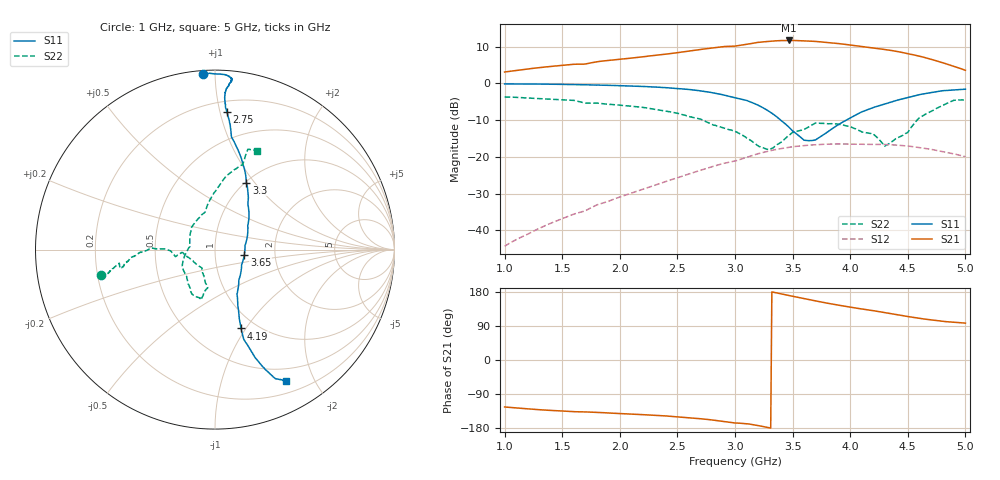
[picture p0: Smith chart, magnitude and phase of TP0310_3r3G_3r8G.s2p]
! Created Fri Jul 02 06:30:30 2021
# hz S ri R 50
! 2 Port Network Data from SP1.SP block
! freq  reS11  imS11  reS21  imS21  reS12  imS12  reS22  imS22
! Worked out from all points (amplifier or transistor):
!   401 points, 1 GHz to 5 GHz, reference 50 ohm
!   highest |S21| = 11.7 dB at 3.47 GHz (marker M1)
!   |S21| within 3 dB of that: 2.575 GHz to 4.41 GHz (1.835 GHz wide, 52.5 % of centre)
!   unconditionally stable (mu >= 1): start of sweep to end of sweep
!   at 1.66 GHz: K = 1.28, MAG = 16.9 dB, |S12| = -35.0 dB
!   at 3 GHz: K = 1.17, MAG = 13.1 dB, |S12| = -21.1 dB
!   at 5 GHz: K = 1.22, MAG = 8.9 dB, |S12| = -20.0 dB
!   S11 on the Smith chart (normalised r, x): 1 GHz: 0.02, +0.93; 2.75 GHz: 0.28, +1.05; 3.3 GHz: 1.01, +0.91; 3.65 GHz: 1.39, -0.09; 4.19 GHz: 0.85, -0.95; 5 GHz: 0.34, -1.62
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1e9  -0.0659 0.9803  -0.7963 -1.184  -0.00607 -0.000702  -0.6363 -0.1393
1.67e9  0.0924 0.9541  -1.332 -1.251  -0.0176 -0.00339  -0.5456 -0.086
1.81e9  0.0918 0.9437  -1.475 -1.323  -0.022 -0.0045  -0.5281 -0.1042
2.34e9  0.0587 0.8832  -2.037 -1.344  -0.0425 -0.00769  -0.4338 -0.0247
2.75e9  0.0663 0.7674  -2.714 -1.18  -0.0694 -0.00525  -0.3004 0.0041
2.9e9  0.0853 0.6905  -3.012 -0.9647  -0.0816 -0.000107  -0.2471 -0.00708
3e9  0.0916 0.6288  -3.115 -0.7669  -0.0875 0.00479  -0.22 -0.0395
3.12e9  0.128 0.5562  -3.363 -0.6643  -0.1003 0.00882  -0.1728 -0.0246
3.2e9  0.1545 0.4813  -3.582 -0.4381  -0.1092 0.0166  -0.1303 -0.0557
3.3e9  0.1751 0.3728  -3.742 -0.0627  -0.1174 0.0295  -0.0728 -0.1015
3.47e9  0.1883 0.1679  -3.773 0.6603  -0.1239 0.054  -0.0501 -0.1903
3.65e9  0.1635 -0.0304  -3.507 1.349  -0.1203 0.0804  -0.0649 -0.2528
3.67e9  0.1587 -0.052  -3.459 1.417  -0.1192 0.0832  -0.0702 -0.2634
3.8e9  0.1328 -0.1705  -3.124 1.803  -0.1111 0.0992  -0.0852 -0.2692
3.92e9  0.1242 -0.26  -2.77 2.045  -0.101 0.1108  -0.1318 -0.2409
4.19e9  0.1454 -0.4395  -1.976 2.299  -0.0749 0.1273  -0.179 -0.0978
4.29e9  0.1579 -0.4923  -1.682 2.361  -0.0658 0.1322  -0.1466 0.00882
4.34e9  0.1729 -0.5195  -1.537 2.371  -0.0591 0.1342  -0.1404 0.0588
4.49e9  0.2194 -0.595  -1.089 2.307  -0.0417 0.1348  -0.0667 0.1997
4.66e9  0.2841 -0.6712  -0.6632 2.113  -0.0221 0.1277  0.0412 0.3829
4.82e9  0.3427 -0.7202  -0.3749 1.832  -0.00713 0.1161  0.1607 0.491
5e9  0.3934 -0.7341  -0.1926 1.492  0.000771 0.1005  0.232 0.5504
